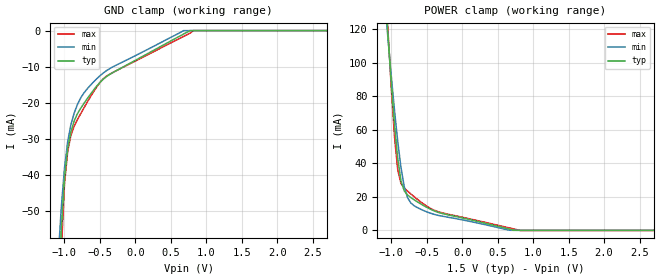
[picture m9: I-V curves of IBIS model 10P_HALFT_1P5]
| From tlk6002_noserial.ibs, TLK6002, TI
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[Model]   10P_HALFT_1P5
Model_type   Input
Polarity   Non-Inverting
Vinh =  0.85
Vinl =  0.65
C_comp   2.108887p   1.924381p   2.428843p
[Model Spec]
Vinh   0.85   0.775   0.925
Vinl   0.65   0.575   0.725
[Temperature Range]   25   125   -40
[Voltage Range]   1.5   1.35   1.65
[POWER_clamp]
-1.5V     431.5mA    358.7mA    512.2mA
-1.091V   144.4mA    136.3mA    154.2mA
-1.045V   115.3mA    113.6mA    118mA
-954.5mV  62.89mA    71.33mA    55.51mA
-909.1mV  42.57mA    52.86mA    35.94mA
-863.6mV  29.45mA    37.4mA     27.95mA
-818.2mV  23.55mA    26.18mA    25.23mA
-772.7mV  21.14mA    19.64mA    23.44mA
-681.8mV  18.34mA    14.76mA    20.19mA
-318.2mV  10.42mA    8.74mA     10.82mA
818.2mV   0A         0A         -106uA
3V        0A         0A         -106uA
[GND_clamp]
-1.5V     -351.3mA   -255.9mA   -467.8mA
-1.091V   -76.16mA   -63.61mA   -90.72mA
-1.045V   -55.4mA    -49.15mA   -61.54mA
-1V       -40.88mA   -38.13mA   -42.53mA
-954.5mV  -32.61mA   -30.72mA   -33.46mA
-909.1mV  -28.01mA   -26.03mA   -28.98mA
-863.6mV  -25.03mA   -22.85mA   -26.45mA
-681.8mV  -18.92mA   -16.18mA   -19.91mA
-500mV    -14.34mA   -12.5mA    -14.38mA
-363.6mV  -12.14mA   -10.54mA   -12.08mA
772.7mV   0A         0A         -692uA
3V        0A         0A         0A
